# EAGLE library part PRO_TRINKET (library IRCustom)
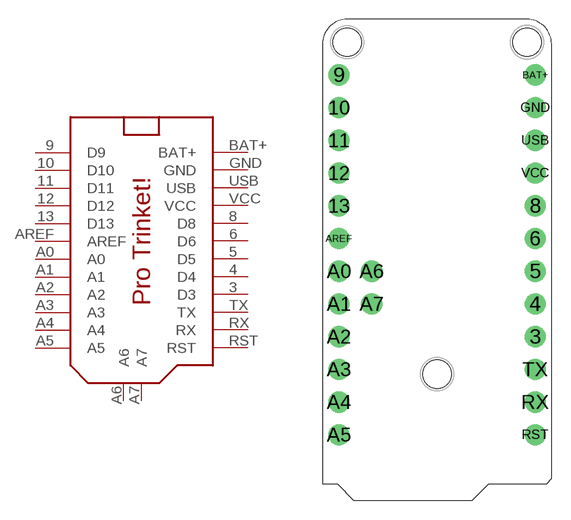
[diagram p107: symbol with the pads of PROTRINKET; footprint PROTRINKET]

Designator prefix -

## PRO_TRINKET  [PROTRINKET]
3  D3
4  D4
5  D5
6  D6
8  D8
9  D9
10  D10
11  D11
12  D12
13  D13
A0  A0
A1  A1
A2  A2
A3  A3
A4  A4
A5  A5
A6  A6  pas
A7  A7  pas
AREF  AREF  pas
BAT+  BAT+  pwr
GND  GND  pwr
RST  RST  pas
RX  RX
TX  TX
USB  USB  pwr
VCC  VCC  pwr

## Footprint PROTRINKET (pad centres in mm)
drill 1.1: 3 7.62,2.921; 4 7.62,5.461; 5 7.62,8.001; 6 7.62,10.541; 8 7.62,13.081; 9 -7.62,23.241; 10 -7.62,20.701; 11 -7.62,18.161; 12 -7.62,15.621; 13 -7.62,13.081; A0 -7.62,8.001; A1 -7.62,5.461; A2 -7.62,2.921; A3 -7.62,0.381; A4 -7.62,-2.159; A5 -7.62,-4.699; A6 -5.08,8.001; A7 -5.08,5.461; AREF -7.62,10.541; BAT+ 7.62,23.241; GND 7.62,20.701; RST 7.62,-4.699; RX 7.62,-2.159; TX 7.62,0.381; USB 7.62,18.161; VCC 7.62,15.621
hole 2.2 at -6.985,25.781
hole 2.2 at 6.985,25.781
hole 2.2 at 0,0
